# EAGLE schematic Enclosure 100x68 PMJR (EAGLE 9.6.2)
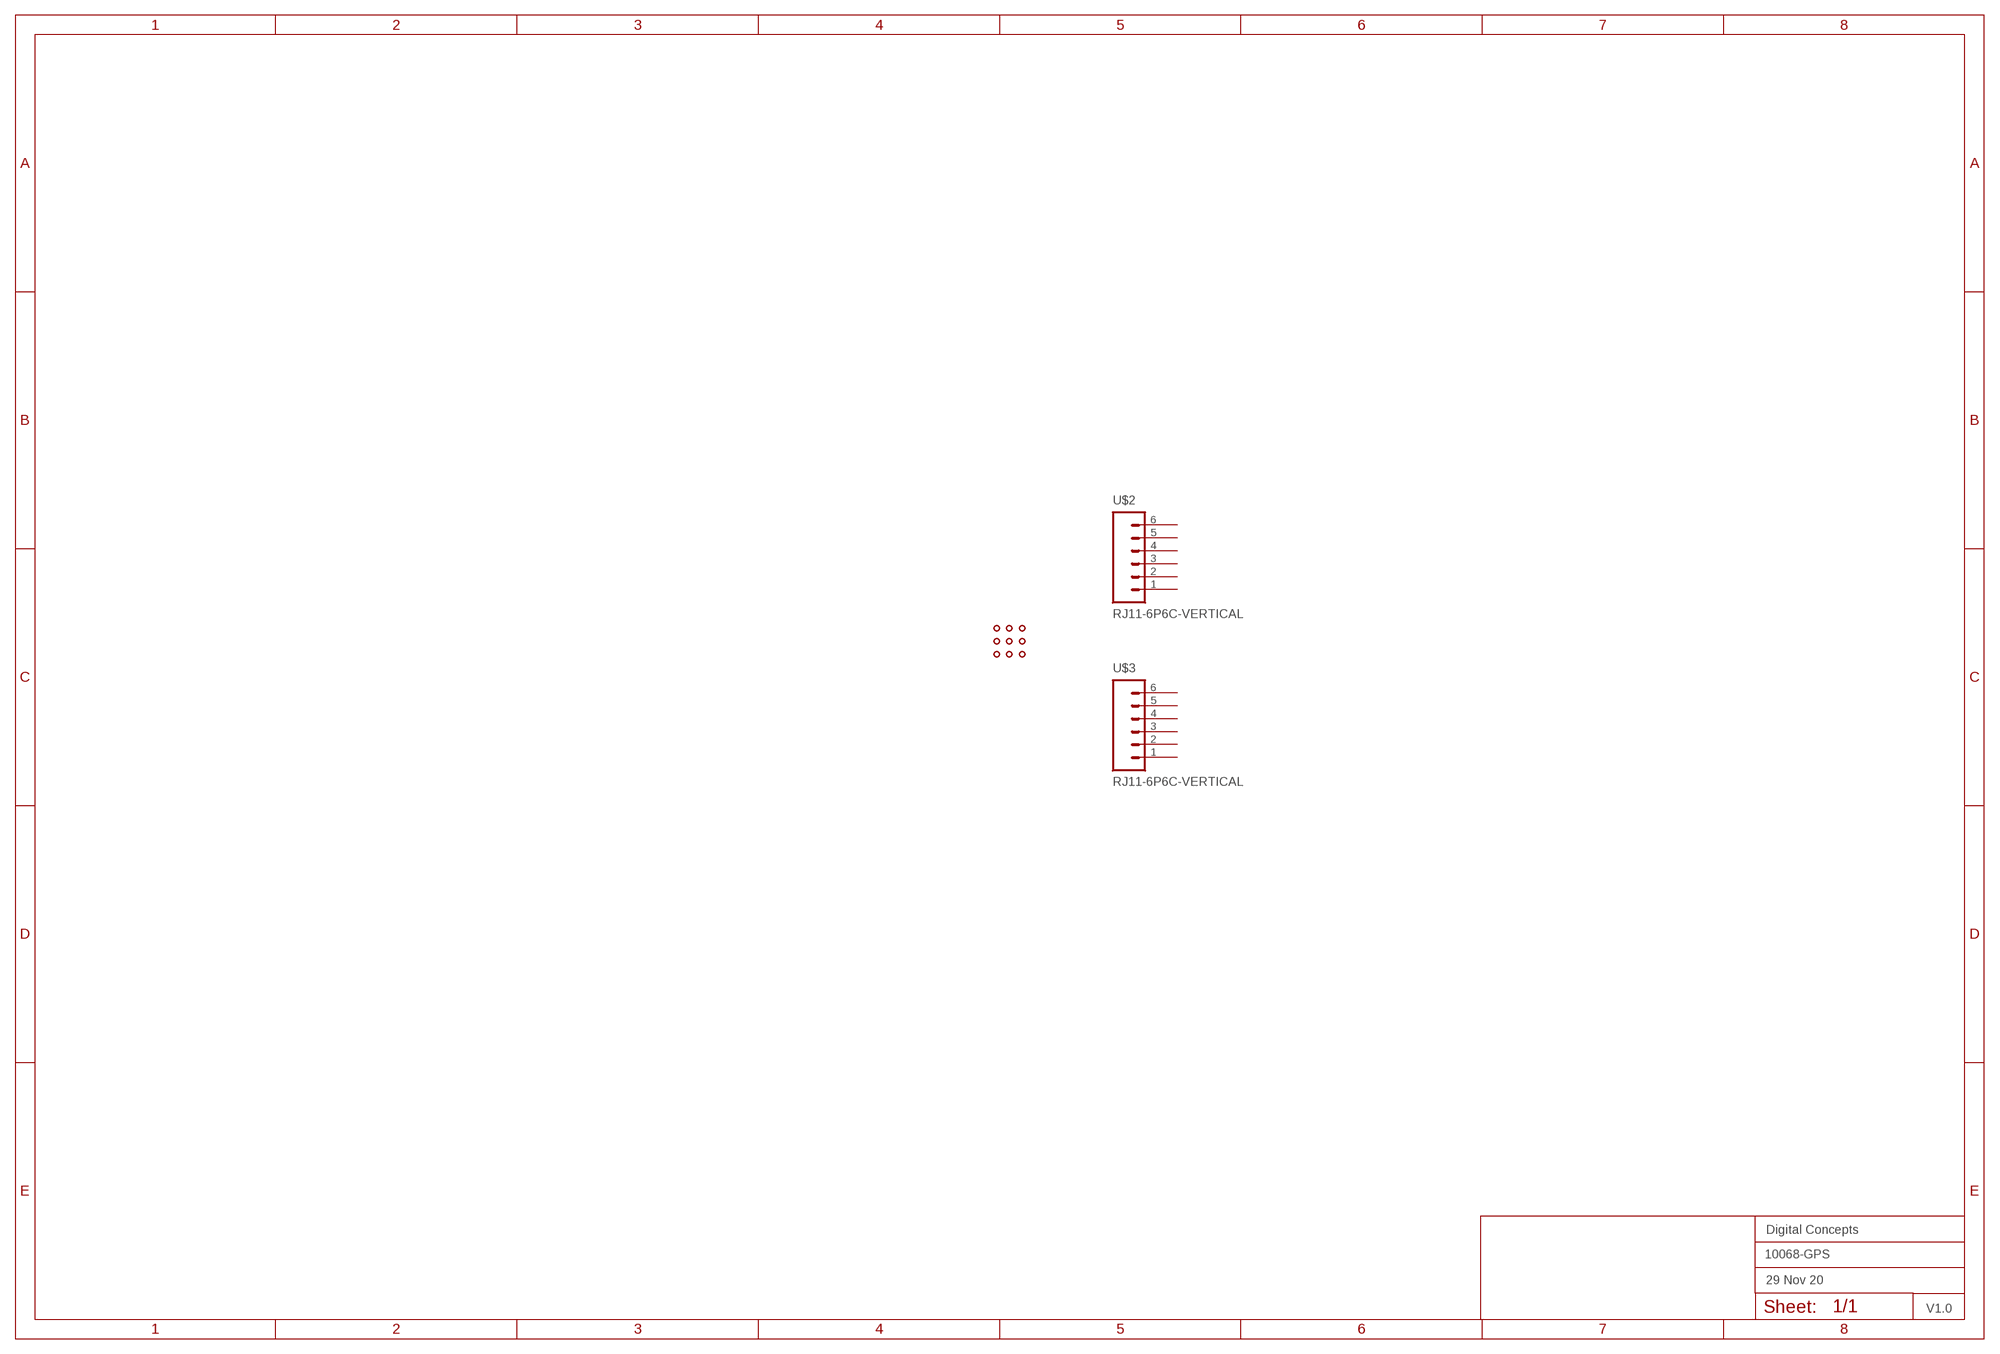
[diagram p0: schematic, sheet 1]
FRAME2 (A3L-LOC): DATE: 29 Nov 20; OWNER: Digital Concepts; TITLE: 10068-GPS; VERSION: V1.0

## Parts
U$1  PROTO-34X22-JST-RJ  [PROTO-34X22-JST-RJ]
U$2  RJ11-6P6C-VERTICAL  [RJ11-6-VERTICAL]
U$3  RJ11-6P6C-VERTICAL  [RJ11-6-VERTICAL]
Unconnected: U$2.1 U$2.2 U$2.3 U$2.4 U$2.5 U$2.6 U$3.1 U$3.2 U$3.3 U$3.4 U$3.5 U$3.6

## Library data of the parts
U$1 = digitalconcepts:PROTO-34X22-JST-RJ: 34 x 22 Prototyping board with JST connector points and space for RJ11 sockets to fit an 100 x 68 enclosure
U$2 U$3 = digitalconcepts:RJ11-6P6C-VERTICAL: RJ11-6P6C-Vertical PCB Socket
